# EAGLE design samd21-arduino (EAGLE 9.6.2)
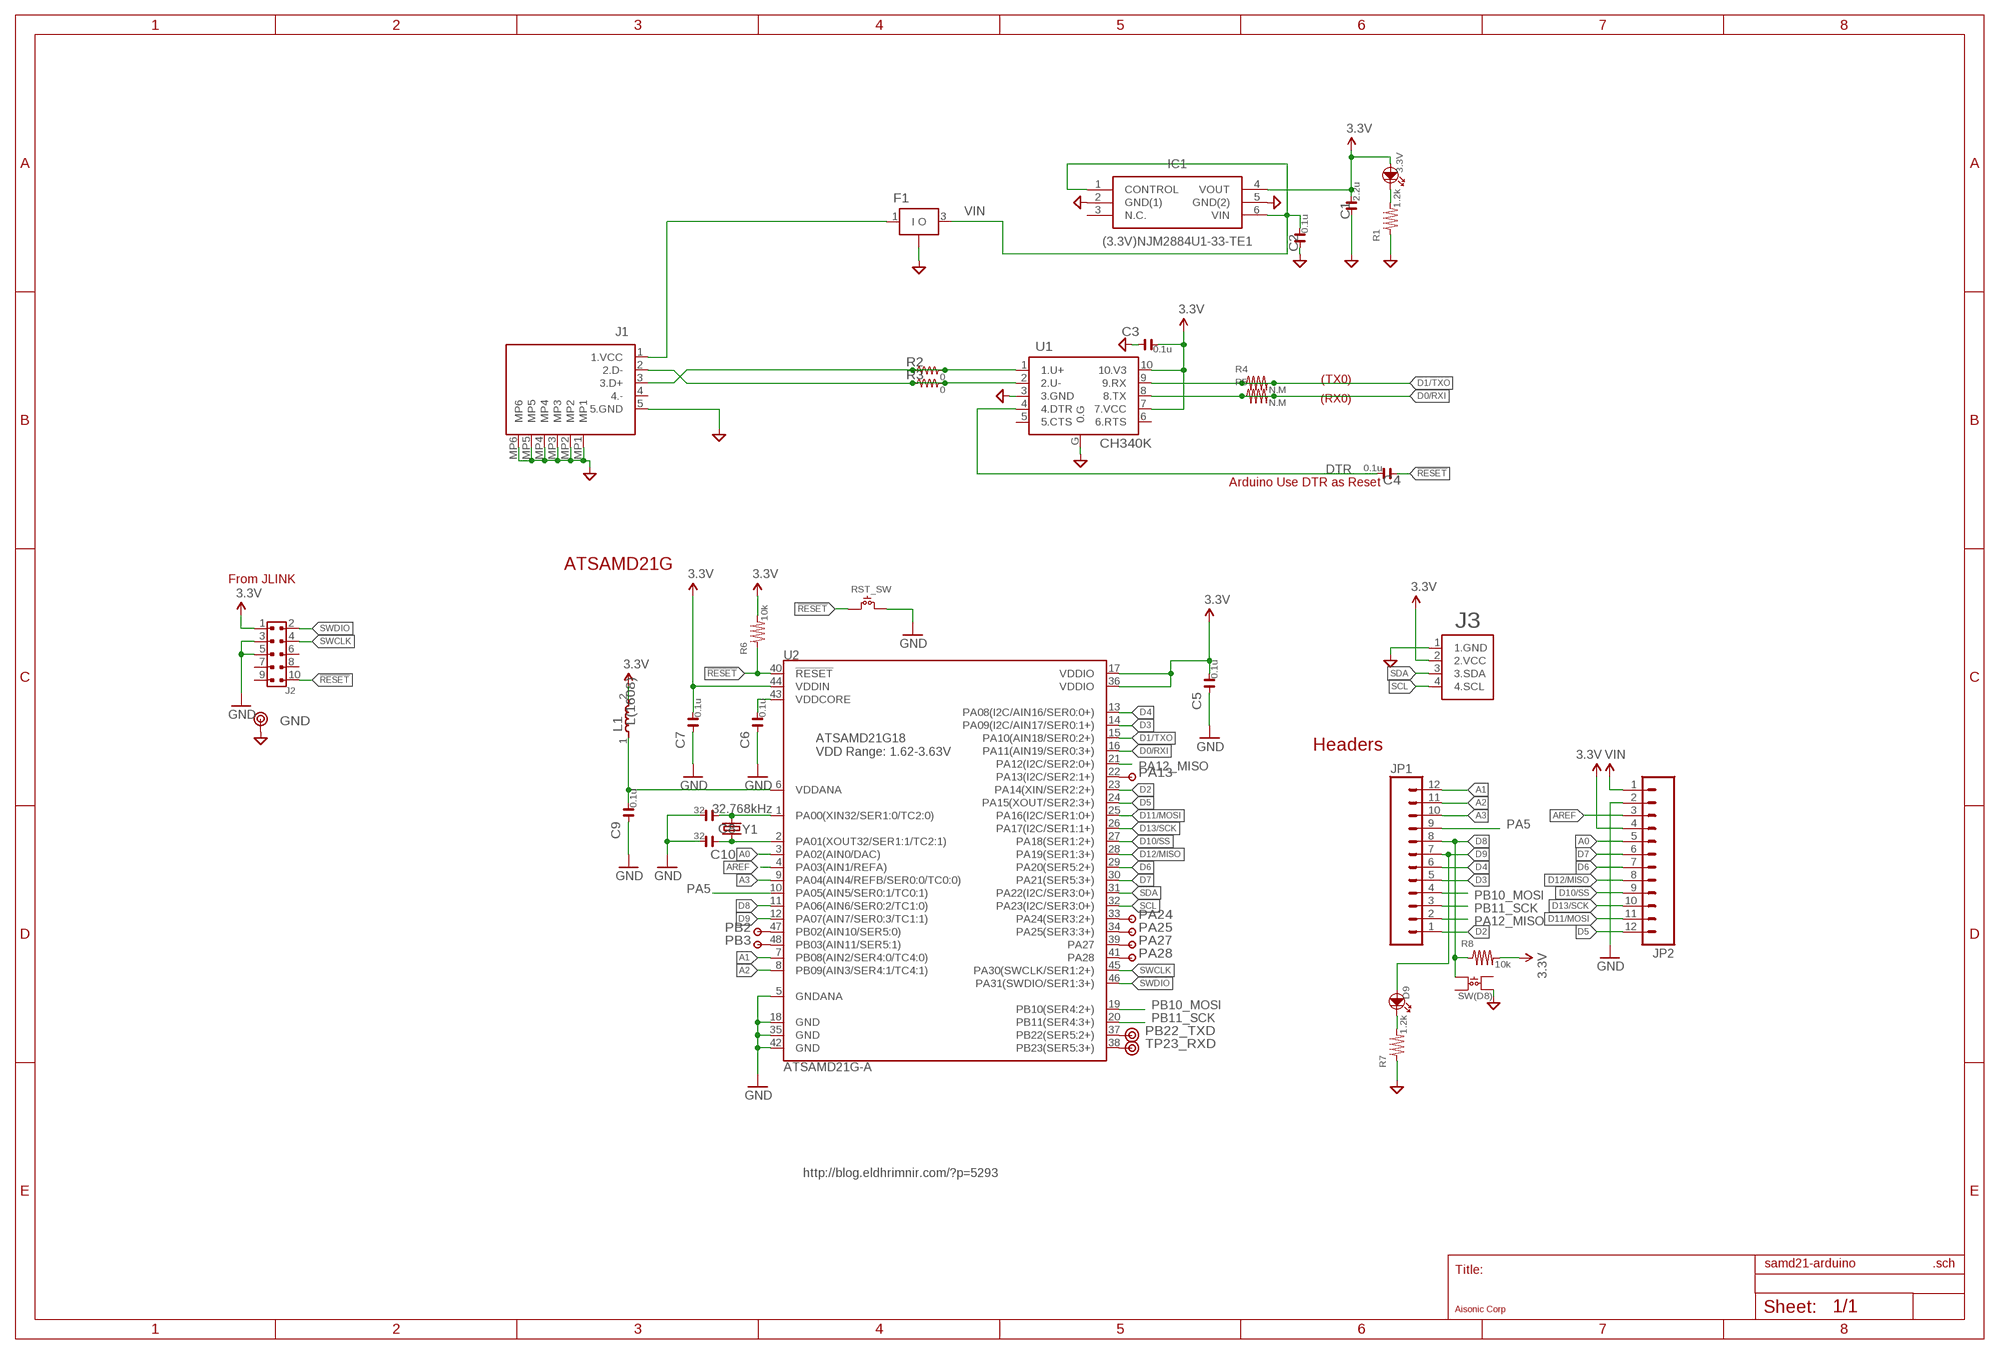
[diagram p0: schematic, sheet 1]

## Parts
3.3V  (PAS)LED[1608]  [1608LED]
C1  2.2u  (PAS)C[1608]  [1608NEW]
C2  0.1u  (PAS)C[1608]  [1608NEW]
C3  0.1u  (PAS)C[1608]  [1608NEW]
C4  0.1u  (PAS)C[1608]  [1608NEW]
C5  0.1u  (PAS)C[1608]  [1608NEW]
C6  0.1u  (PAS)C[1608]  [1608NEW]
C7  0.1u  (PAS)C[1608]  [1608NEW]
C8  32  (PAS)C[1608]  [1608NEW]
C9  0.1u  (PAS)C[1608]  [1608NEW]
C10  32  (PAS)C[1608]  [1608NEW]
D9  (PAS)LED[1608]  [1608LED]
F1  (EMI-FIL)NFM21PC(2012)  [EMIFILL]
FRAME1  (!)A3L-LOC  [D3LOGO-PAC]
GND  TP-HOLE  [TP-HOLE]
IC1  (3.3V)NJM2884U1-33-TE1  [SOT-89-5-1]
J1  (USB)USB-MICRO(ZX62-B-5PA_33)  [ZX62B5PA33]
J2  ARMJTAG10PINSTRAIT  [JTAG_HALFPITCH]
J3  GROVE-I2C  [GROVE-4P]
JP1  M12NO_SILK  [1X12_NO_SILK]
JP2  M12NO_SILK  [1X12_NO_SILK]
L1  L(1608)  [1608NEW]
PA13  TP  [TP-SQUARE]
PA24  TP  [TP-SQUARE]
PA25  TP  [TP-SQUARE]
PA27  TP  [TP-SQUARE]
PA28  TP  [TP-SQUARE]
PB2  TP  [TP-SQUARE]
PB3  TP  [TP-SQUARE]
PB22_TXD  TP-HOLE  [TP-HOLE]
R1  1.2k  (PAS)R[1608]  [1608NEW]
R2  0  R(1005)  [1005]
R3  0  R(1005)  [1005]
R4  N.M  (PAS)R[1608]  [1608NEW]
R5  N.M  (PAS)R[1608]  [1608NEW]
R6  10k  (PAS)R[1608]  [1608NEW]
R7  1.2k  (PAS)R[1608]  [1608NEW]
R8  10k  (PAS)R[1608]  [1608NEW]
RST_SW  (SW)RST_SW(TVAF06)  [TVAF06]
SW(D8)  (SW)USER_SW(AKIDUKI)  [SKRPACE010-PAC]
TP23_RXD  TP-HOLE  [TP-HOLE]
U1  CH340K  (USB)CH340K  [ESSOP10]
U2  ATSAMD21G-A  [TQFP-48]
Y1  32.768kHz  CRYSTAL3.2X1.5MM  [CRYSTAL-SMD-3.2X1.5MM]

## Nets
3.3V: 3.3V.1(+) C1.2 C3.2 C5.2 C7.2 IC1.4(VOUT) J2.1 J3.2(2.VCC) JP2.4 L1.2 R6.2 R8.2 U1.7(7.VCC) U1.10(10.V3) U2.17(VDDIO) U2.36(VDDIO) U2.44(VDDIN)
!RESET: C4.1 J2.10 R6.1 RST_SW.P$1 U2.40(!RESET!)
A0: JP2.5 U2.3(PA02(AIN0/DAC))
A1: JP1.12 U2.7(PB08(AIN2/SER4:0/TC4:0))
A2: JP1.11 U2.8(PB09(AIN3/SER4:1/TC4:1))
A3: JP1.10 U2.9(PA04(AIN4/REFB/SER0:0/TC0:0))
AREF: JP2.3 U2.4(PA03(AIN1/REFA))
D0/RXI: R5.1 R5.2 U1.8(8.TX) U2.16(PA11(AIN19/SER0:3+))
D1/TXO: R4.1 R4.2 U1.9(9.RX) U2.15(PA10(AIN18/SER0:2+))
D2: JP1.1 U2.23(PA14(XIN/SER2:2+))
D3: JP1.5 U2.14(PA09(I2C/AIN17/SER0:1+))
D4: JP1.6 U2.13(PA08(I2C/AIN16/SER0:0+))
D5: JP2.12 U2.24(PA15(XOUT/SER2:3+))
D6: JP2.7 U2.29(PA20(SER5:2+))
D7: JP2.6 U2.30(PA21(SER5:3+))
D8: JP1.8 R8.1 SW(D8).1 U2.11(PA06(AIN6/SER0:2/TC1:0))
D9: D9.1(+) JP1.7 U2.12(PA07(AIN7/SER0:3/TC1:1))
D10/SS: JP2.9 U2.27(PA18(SER1:2+))
D11/MOSI: JP2.11 U2.25(PA16(I2C/SER1:0+))
D12/MISO: JP2.8 U2.28(PA19(SER1:3+))
D13/SCK: JP2.10 U2.26(PA17(I2C/SER1:1+))
DTR: C4.2 U1.4(4.DTR)
GND: C1.1 C2.1 C3.1 C5.1 C6.1 C7.1 C8.2 C9.1 C10.2 F1.2(G) GND.1 IC1.2(GND(1)) IC1.5(GND(2)) J1.5(5.GND) J1.MP1 J1.MP2 J1.MP3 J1.MP4 J1.MP5 J1.MP6 J2.3 J2.5 J3.1(1.GND) JP2.2 R1.1 R7.1 RST_SW.P$2 SW(D8).4 U1.3(3.GND) U1.G(0.G) U2.5(GNDANA) U2.18(GND) U2.35(GND) U2.42(GND)
N$1: PA24.1 U2.33(PA24(SER3:2+))
N$2: C8.1 U2.1(PA00(XIN32/SER1:0/TC2:0)) Y1.P$2
N$3: PA25.1 U2.34(PA25(SER3:3+))
N$4: C10.1 U2.2(PA01(XOUT32/SER1:1/TC2:1)) Y1.P$1
N$5: PA27.1 U2.39(PA27)
N$6: PA28.1 U2.41(PA28)
N$7: D9.2(-) R7.2
N$9: PB22_TXD.1 U2.37(PB22(SER5:2+))
N$10: TP23_RXD.1 U2.38(PB23(SER5:3+))
N$11: PA13.1 U2.22(PA13(I2C/SER2:1+))
N$14: 3.3V.2(-) R1.2
N$15: J1.3(3.D+) R2.1 R2.2 U1.1(1.U+)
N$16: J1.2(2.D-) R3.1 R3.2 U1.2(2.U-)
N$17: PB3.1 U2.48(PB03(AIN11/SER5:1))
N$18: PB2.1 U2.47(PB02(AIN10/SER5:0))
PA5: JP1.9 U2.10(PA05(AIN5/SER0:1/TC0:1))
PA12_MISO: JP1.2 U2.21(PA12(I2C/SER2:0+))
PB10_MOSI: JP1.4 U2.19(PB10(SER4:2+))
PB11_SCK: JP1.3 U2.20(PB11(SER4:3+))
SCL: J3.4(4.SCL) U2.32(PA23(I2C/SER3:0+))
SDA: J3.3(3.SDA) U2.31(PA22(I2C/SER3:0+))
SWCLK: J2.4 U2.45(PA30(SWCLK/SER1:2+))
SWDIO: J2.2 U2.46(PA31(SWDIO/SER1:3+))
VBUS5V1: F1.1(I) J1.1(1.VCC)
VDDANA: C9.2 L1.1 U2.6(VDDANA)
VDDCORE: C6.2 U2.43(VDDCORE)
VIN: C2.2 F1.3(O) IC1.1(CONTROL) IC1.6(VIN) JP2.1
Unconnected: IC1.3(N.C.) J1.4(4.-) J2.6 J2.7 J2.8 J2.9 SW(D8).2 SW(D8).3 U1.5(5.CTS) U1.6(6.RTS)

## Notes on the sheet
- (TX0)
- (RX0)
- Arduino Use DTR as Reset
- ATSAMD21G
- From JLINK
- Headers
- ATSAMD21G18
  VDD Range: 1.62-3.63V
- http://blog.eldhrimnir.com/?p=5293

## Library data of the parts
3.3V D9 = myEagleParts8:(PAS)LED[1608]
C1-C10 = myEagleParts8:(PAS)C[1608]
F1 = myEagleParts8:(EMI-FIL)NFM21PC(2012)
FRAME1 = myEagleParts8:(!)A3L-LOC: FRAME
GND PB22_TXD TP23_RXD = myEagleParts8:TP-HOLE
IC1 = myEagleParts8:(3.3V)NJM2884U1-33-TE1: Low Dropout Voltage Regulator New Japan Radio NJM2884U1-33-TE1, LDO Voltage Regulator, 0.65A, 3.3 V 1%, 5-Pin SOT-89 Source: Datasheet; DESCRIPTION: Low Dropout Voltage Regulator New Japan Radio NJM2884U1-33-TE1, LDO Voltage Regulator, 0.65A, 3.3 V 1%, 5-Pin SOT-89; HEIGHT: mm; MANUFACTURER_NAME: New Japan Radio; MANUFACTURER_PART_NUMBER: NJM2884U1-33-TE1; RS_PART_NUMBER: 7139366P; SUPPLIER_NAME: RS
J1 = myEagleParts8:(USB)USB-MICRO(ZX62-B-5PA_33): USB Connectors MICRO B RECEPT RA SMT BTTM MNT Source: Datasheet; DESCRIPTION: USB Connectors MICRO B RECEPT RA SMT BTTM MNT; HEIGHT: 3mm; MANUFACTURER_NAME: Hirose; MANUFACTURER_PART_NUMBER: ZX62-B-5PA(33); RS_PART_NUMBER: 1362267; RS_PRICE-STOCK: http://uk.rs-online.com/web/p/products/1362267
J2 = myEagleParts8:ARMJTAG10PIN
J3 = myEagleParts8:GROVE-I2C
JP1 JP2 = SparkFun-Connectors:M12: Header 12 Standard 12-pin 0.1" header. Use with straight break away headers (SKU : PRT-00116), right angle break away headers (PRT-00553), swiss pins (PRT-00743), machine pins (PRT-00117), and female headers (PRT-00115).
L1 = myEagleParts8:L(1608)
PA13 PA24 PA25 PA27 PA28 PB2 PB3 = myEagleParts8:TP
R1 R4-R8 = myEagleParts8:(PAS)R[1608]
R2 R3 = myEagleParts8:R(1005)
RST_SW = myEagleParts8:(SW)RST_SW(TVAF06)
SW(D8) = myEagleParts8:(SW)USER_SW(AKIDUKI): http://akizukidenshi.com/catalog/g/gP-06185/
U1 = myEagleParts8:(USB)CH340K
U2 = samd21-temp:ATSAMD21G: Atmel SAMD21G SMART ARM-Based Microcontroller The Atmel ® | SMART ™ SAM D21 is a series of low-power microcontrollers using the 32-bit ARM ® Cortex ® -M0+ processor, and ranging from 32- to 64-pins with up to 256KB Flash and 32KB of SRAM. The SAM D21 devices operate at a maximum frequency of 48MHz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; PROD_ID: IC-13064
Y1 = samd21-temp:CRYSTAL: Various standard crystals. Proven footprints.; PROD_ID: XTAL-13062

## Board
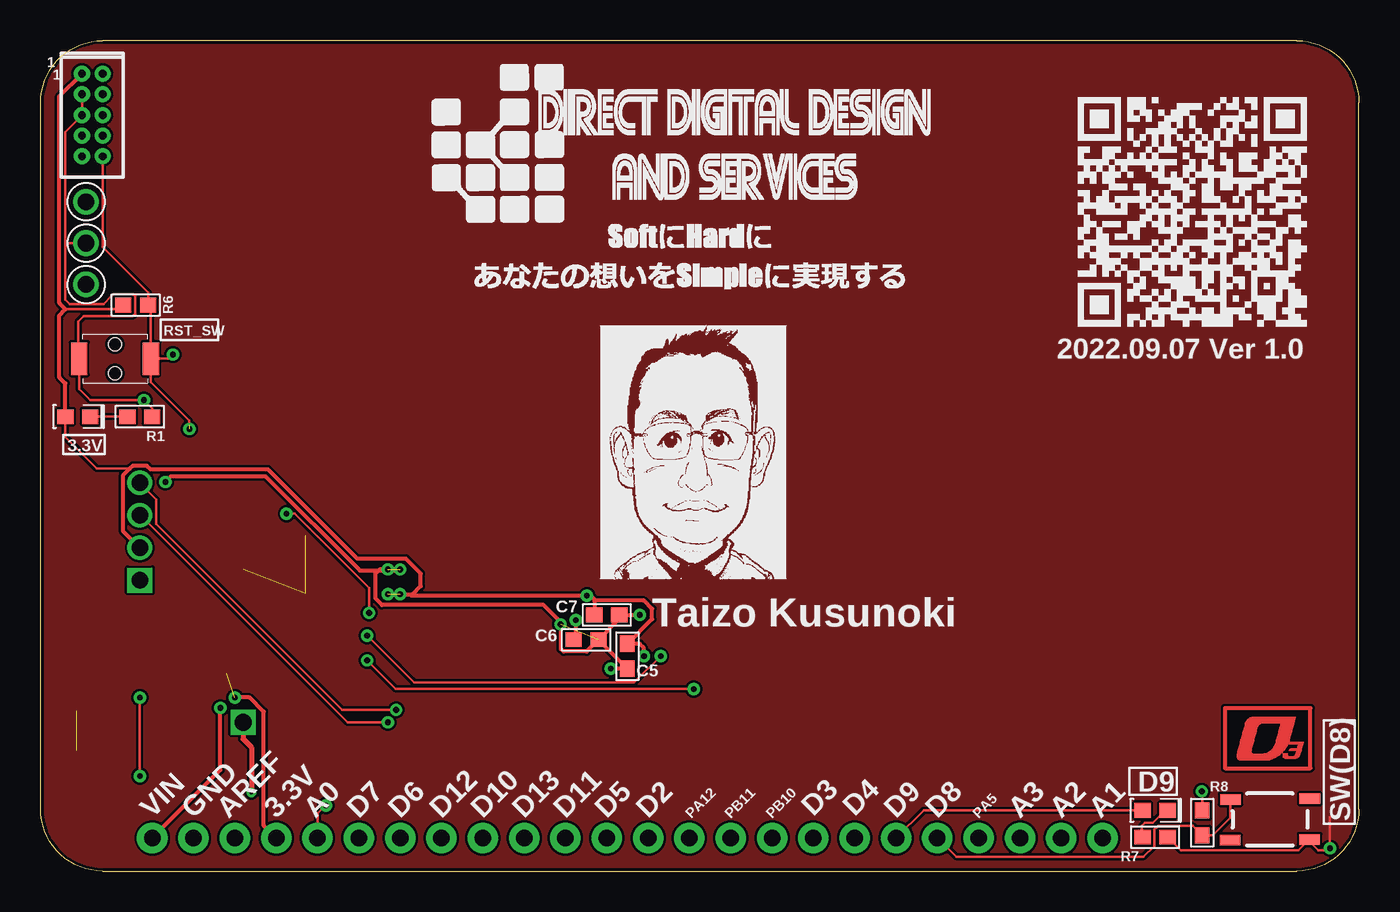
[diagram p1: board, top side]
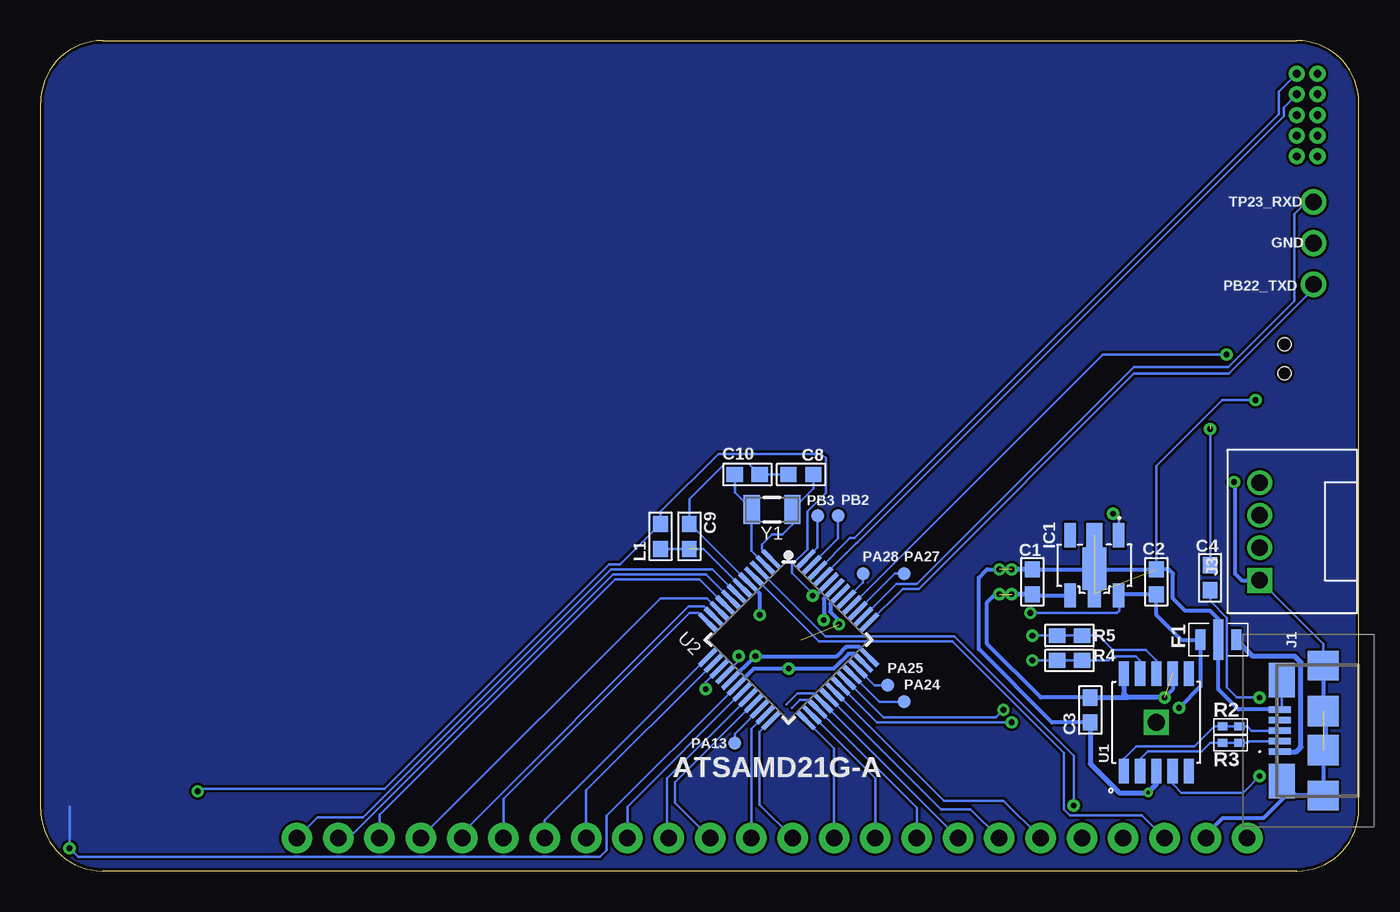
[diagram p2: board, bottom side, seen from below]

Size 81.03 x 51.05 mm. Coordinates in mm from the lower left corner, seen from the top.
Outline: 0,3.56 0,47.24 arc-90 3.81,51.05 77.22,51.05 arc-90 81.03,47.24 81.03,3.81 arc-90 77.22,0 3.81,0 arc-90 0,3.81
Copper layers (1*16): Top 0.035mm / dielectric 1.5mm / Bottom 0.035mm
Design rules "PCBGoGo": minimum track width 6mil, minimum drill 0.2mm, track to track 6mil, track to pad 6mil, pad to pad 6mil, via to via 6mil, smd to smd 6mil, copper to edge 0.2mm, drill to drill 6mil, minimum pad ring 10mil, minimum via ring 8mil, stop-mask expansion 4mil, vias tented up to drill 0mil, thermal gap 10mil

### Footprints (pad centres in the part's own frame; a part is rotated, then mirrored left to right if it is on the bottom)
1608LED = smd 1 x 0.9: 1 -0.766,0; 2 0.766,0
1608NEW = smd 1 x 0.9: 1 -0.766,0; 2 0.766,0
EMIFILL = smd 0.6 x 1.25: 1 -1.1,0; 3 1.1,0 | smd 0.6 x 2.5: 2 0,0
TP-HOLE = drill 1.016 pad 1.575: 1 0,0
SOT-89-5-1 = smd 0.7 x 1.5: 1 -1.5,-1.85; 3 1.5,-1.85; 4 1.5,1.85; 6 -1.5,1.85 | smd 1 x 1.5: 2 0,-1.85 | smd 0.8 x 1.5: 5 0,1.85 | smd 1.5 x 2.6: 7 0,0.2
ZX62B5PA33 = smd 0.4 x 1.35: 1 -1.3,2.325; 2 -0.65,2.325; 3 0,2.325; 4 0.65,2.325; 5 1.3,2.325 | smd 1.8 x 1.9: MP1 -4,-0.35; MP2 4,-0.35 | smd 2.1 x 1.6: MP3 -3.1,2.2; MP4 3.1,2.2 | smd 1.9 x 1.9: MP5 -1.2,-0.35; MP6 1.2,-0.35
JTAG_HALFPITCH = drill 0.483 pad 0.61: 1 0,0; 2 1.27,0; 3 0,-1.27; 4 1.27,-1.27; 5 0,-2.54; 6 1.27,-2.54; 7 0,-3.81; 8 1.27,-3.81; 9 0,-5.08; 10 1.27,-5.08
GROVE-4P = drill 1.016 square: 1 6,0 | drill 1.016: 2 4,0; 3 2,0; 4 0,0
1X12_NO_SILK = drill 1.016 pad 1.88: 1 0,0; 2 2.54,0; 3 5.08,0; 4 7.62,0; 5 10.16,0; 6 12.7,0; 7 15.24,0; 8 17.78,0; 9 20.32,0; 10 22.86,0; 11 25.4,0; 12 27.94,0
TP-SQUARE = smd 0.8 x 0.8: 1 0,0
1005 = smd 0.6 x 0.5: 1 -0.508,0; 2 0.519,0
TVAF06 = smd 2 x 1: P$1 0,2.2; P$2 0,-2.2 | hole 0.8: -0.9,0; 0.9,0
SKRPACE010-PAC = smd 1.27 x 0.635: 1 -2.427,1.227; 2 -2.45,-1.277; 3 2.45,1.277; 4 2.427,-1.227
ESSOP10 = smd 1.5 x 0.635: 1 -3,2; 2 -3,1; 3 -3,0; 4 -3,-1; 5 -3,-2; 6 3,-2; 7 3,-1; 8 3,0; 9 3,1; 10 3,2 | drill 1.016 square: G 0,0
TQFP-48 = smd 1.5 x 0.28: 1 -4.25,2.75; 2 -4.25,2.25; 3 -4.25,1.75; 4 -4.25,1.25; 5 -4.25,0.75; 6 -4.25,0.25; 7 -4.25,-0.25; 8 -4.25,-0.75; 9 -4.25,-1.25; 10 -4.25,-1.75; 11 -4.25,-2.25; 12 -4.25,-2.75; 25 4.25,-2.75; 26 4.25,-2.25; 27 4.25,-1.75; 28 4.25,-1.25; 29 4.25,-0.75; 30 4.25,-0.25; 31 4.25,0.25; 32 4.25,0.75; 33 4.25,1.25; 34 4.25,1.75; 35 4.25,2.25; 36 4.25,2.75 | smd 0.28 x 1.5: 13 -2.75,-4.25; 14 -2.25,-4.25; 15 -1.75,-4.25; 16 -1.25,-4.25; 17 -0.75,-4.25; 18 -0.25,-4.25; 19 0.25,-4.25; 20 0.75,-4.25; 21 1.25,-4.25; 22 1.75,-4.25; 23 2.25,-4.25; 24 2.75,-4.25; 37 2.75,4.25; 38 2.25,4.25; 39 1.75,4.25; 40 1.25,4.25; 41 0.75,4.25; 42 0.25,4.25; 43 -0.25,4.25; 44 -0.75,4.25; 45 -1.25,4.25; 46 -1.75,4.25; 47 -2.25,4.25; 48 -2.75,4.25
CRYSTAL-SMD-3.2X1.5MM = smd 1 x 1.8: P$1 -1.25,0; P$2 1.25,0

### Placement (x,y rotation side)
3.3V  2.29,27.94 0 top
C1  20.07,17.78 270 bottom
C2  12.45,17.78 270 bottom
C3  16.51,9.91 90 bottom
C4  9.14,18.03 270 bottom
C5  36.07,13.21 90 top
C6  33.53,14.22 180 top
C7  34.8,15.75 180 top
C8  34.29,24.38 180 bottom
C9  41.15,20.57 270 bottom
C10  37.59,24.38 0 bottom
D9  68.5,3.73 0 top
F1  8.64,14.22 180 bottom
FRAME1  72.8,6.38 0 top
GND  2.79,38.61 0 top
IC1  16.26,18.8 180 bottom
J1  2.54,8.64 90 bottom
J2  2.54,49.02 0 top
J3  6.1,23.88 270 bottom
JP1  37.34,2.03 0 top
JP2  6.86,2.03 0 top
L1  42.93,20.57 90 bottom
PA13  38.35,7.87 0 bottom
PA24  27.94,10.41 0 bottom
PA25  28.96,11.43 0 bottom
PA27  27.94,18.29 0 bottom
PA28  30.48,18.29 0 bottom
PB2  32,21.84 0 bottom
PB3  33.27,21.84 0 bottom
PB22_TXD  2.79,36.07 0 top
R1  6.1,27.94 180 top
R2  7.87,8.89 0 bottom
R3  7.87,7.87 0 bottom
R4  17.78,12.95 180 bottom
R5  17.78,14.48 180 bottom
R6  5.84,34.8 180 top
R7  68.5,2.08 180 top
R8  71.4,2.97 90 top
RST_SW  4.57,31.5 270 top
SW(D8)  75.56,3.17 0 top
TP23_RXD  2.79,41.15 0 top
U1  12.45,9.14 90 bottom
U2  35.05,14.22 315 bottom
Y1  36.07,22.23 0 bottom

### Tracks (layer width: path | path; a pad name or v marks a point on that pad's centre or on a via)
3.3V  (via drill 0.35 pad 0.3)  (2 unrouted)
  Top 0.152: R6.2 4.82,34.54 1.52,34.54 | 3.3V.1 1.52,26.67 3.46,24.74 5.49,24.74 | v71.37,4.9 71.4,4.88 R8.2
  Top 0.254: 34.03,16.64 34.03,16.7 33.73,17 33.66,17 v33.58,16.93 33.49,16.93 33.48,16.94 22.78,16.94 22.86,17.02 | 34.03,16.64 C7.2 | v37.08,13.21 37.08,13.72 36.83,13.97 C5.2 37.59,15.5 37.59,16.13 37.08,16.64 34.03,16.64 | J2.1 1.14,47.62 1.14,34.92 1.52,34.54 1.14,34.16 1.14,30.35 1.52,29.98 3.3V.1 | JP2.4 13.72,2.79 13.72,9.79 12.84,10.67 v11.94,10.67 | v21.34,17.02 22.86,17.02 | 22.86,17.02 23.37,17.53 23.37,18.29 22.46,19.2 19.48,19.2 13.98,24.69 6.75,24.69 6.53,24.92 5.67,24.92 5.49,24.74 5.05,24.31 5.05,20.92 J3.2
  Bottom 0.152: 33.58,17.07 v33.58,16.93 | 33.58,17.07 34.85,18.34 34.85,18.84 33.9,19.78 33.9,22.1 32.77,23.24 32.77,25.4 33.02,25.65 39.37,25.65 42.93,22.1 L1.2 45.42,18.85 46.1,18.85 59.89,5.05 71.22,5.05 v71.37,4.9 | 33.58,17.07 33.53,17.02
  Bottom 0.254: U2.44 33.32,17.02 33.53,17.02 | U2.17 37.13,13.21 v37.08,13.21 32.09,13.21 31.52,13.77 30.71,13.77 U2.36 | C1.2 20,16.95 IC1.4 | C3.2 19.56,10.67 22.86,13.97 22.86,16.51 22.36,17.01 v22.09,17.01 | U1.7 11.45,11.16 v11.93,10.67
  Bottom 0.305: C3.2 14.22,10.67 | v11.93,10.67 14.22,10.67 | U1.10 14.45,10.89 14.22,10.67 | C1.2 v22.09,17.01 v22.1,17.02
!RESET  (via drill 0.35 pad 0.3)  (1 unrouted)
  Top 0.152: v8.13,31.75 7.87,31.5 RST_SW.P$1 | RST_SW.P$1 6.77,34.38 6.6,34.54 R6.1 | R6.1 | J2.10 3.81,38.35 6.6,35.56 R6.1 | RST_SW.P$1 6.77,30.06 9.14,27.69 v9.14,27.18
  Bottom 0.152: U2.40 15.75,31.75 v8.13,31.75 | 9.14,27.43 C4.1
A0  (via drill 0.35 pad 0.3)
  Top 0.152: JP2.5 17.02,3.56 17.5,4.04 v17.53,4.04
  Bottom 0.152: U2.3 32.78,14.43 24.87,14.43 17.53,7.08 v17.53,4.04
A1
  Bottom 0.152: U2.7 39.72,18.54 45.97,18.54 61.21,3.3 64.01,3.3 JP1.12
A2
  Bottom 0.152: U2.8 40.13,18.24 45.85,18.24 62.05,2.03 JP1.11
A3
  Bottom 0.152: U2.9 40.53,17.93 45.72,17.93 60.2,3.46 JP1.10
AREF
  Bottom 0.152: U2.4 33.18,14.12 25,14.12 18.13,7.26 18.13,3.78 17.78,3.43 13.34,3.43 JP2.3
BETA_L1
  Top 0.152: 79.25,1.27 79.25,3.3
  pour Top: -2.54,53.34 83.82,53.34 83.82,-2.54 -2.54,-2.54
BETA_L2
  Bottom 0.152: 79.25,1.27 79.25,3.94
  pour Bottom: -5.08,55.88 86.36,55.88 86.36,-5.08 -5.08,-5.08
D0/RXI  (via drill 0.35 pad 0.3)
  Top 0.152: v20.07,14.48 22.96,11.59 36.49,11.59 38.11,13.21 v38.11,13.22
  Bottom 0.152: U1.8 12.45,12.95 13.08,13.59 15.11,13.59 16,14.48 R5.1 R5.2 v20.07,14.48 | v38.11,13.22 38.1,13.21 38.1,12.94 U2.16
D1/TXO  (via drill 0.35 pad 0.3)
  Top 0.152: v40.15,11.19 21.83,11.19 v20.07,12.95
  Bottom 0.152: U1.9 13.45,12.94 13.72,13.21 15.11,13.21 15.37,12.95 R4.1 R4.2 v20.07,12.95 | U2.15 40.15,11.6 v40.15,11.19
D2
  Bottom 0.152: U2.23 37.34,8.76 JP1.1
D3
  Bottom 0.152: JP1.5 47.5,4.96 U2.14
D4
  Bottom 0.152: JP1.6 50.04,3.13 U2.13
D5
  Bottom 0.152: U2.24 36.83,8.56 36.83,4.06 JP2.12
D6
  Bottom 0.152: U2.29 25.7,3.81 23.88,3.81 JP2.7
D7
  Bottom 0.152: U2.30 25.5,4.32 21.84,4.32 JP2.6
D8
  Top 0.152: SW(D8).1 73.14,3.29 72.06,2.21 R8.1 70.81,2.79 68.7,2.79 68.47,2.56 68.47,1.54 67.79,0.86 56.29,0.86 JP1.8
  Bottom 0.152: U2.11 40.27,16.26 41.2,16.26 55.12,2.34 JP1.8
D9
  Top 0.152: JP1.7 54.28,3.73 D9.1
  Bottom 0.152: U2.12 40.59,15.88 41.15,15.88 52.58,4.45 JP1.7
D10/SS
  Bottom 0.152: 34.85,10.03 34.34,10.54 33.84,10.54 U2.27 27.18,3.88 JP2.9
D11/MOSI
  Bottom 0.152: JP2.11 32.26,7.54 U2.25
D12/MISO
  Bottom 0.152: 35.18,10.26 34.52,10.92 33.52,10.92 U2.28 24.64,2.04 JP2.8
D13/SCK
  Bottom 0.152: U2.26 29.72,5.71 JP2.10
DTR  (via drill 0.35 pad 0.3)
  Top 0.152: v6.1,5.84 v6.1,10.67
  Bottom 0.152: U1.4 11.45,5.35 10.92,4.83 7.11,4.83 v6.1,5.84 | 8.89,17.27 C4.2 9.14,16.61 8.11,15.57 8.11,11.28 7.49,10.67 v6.1,10.67
GND  (via drill 0.2 pad 0.3, 0.35 pad 0.3)  (5 unrouted)
  Top 0.152: J2.3 J2.5 1.5,45.44 1.5,38.35 | v6.35,28.96 3.05,28.96 2.37,29.63 RST_SW.P$2 2.32,31.55 2.32,33.78 2.66,34.12 5.67,34.12 5.8,34.25 5.8,35.34 5.67,35.48 4.48,35.48 4.35,35.34 3.86,34.85 1.78,34.85 1.5,35.13 1.5,38.35 | v6.35,28.96 6.86,28.44 R1.1 | GND.1 1.75,38.61 1.5,38.35 | v6.35,28.96 | v79.25,1.4 79.12,1.27 78.54,1.27 77.99,1.82 SW(D8).4 77.31,1.27 70.08,1.27 R7.1
  Top 0.254: C6.1 35.56,15.49 C7.1 v36.83,15.75 | C6.1 C5.1 v35.06,12.44 v35.05,12.45 | v7.67,23.92 8.03,24.29 13.81,24.29 19.62,18.48 22.04,18.48 v22.1,18.54 20.83,18.54 20.57,18.29 20.57,16.76 20.98,16.36 30.92,16.36 31.98,15.3 31.98,13.66 32.15,13.49 33.56,13.49 C6.1
  Top 0.305: U1.G 12.45,8.13 12.95,7.62 v12.95,4.83
  Bottom 0.152: C8.2 C10.2 37.51,25.06 38.95,25.06 41.15,22.87 C9.1 41.11,21.34 U2.5 | J1.MP4 4.74,10.06 J1.5 | C2.1 12.45,24.89 8.38,28.96 v6.35,28.96 | 2.19,12.45 2.19,13.97 J3.1 | IC1.5 16.26,17.07 | U2.18 46.23,3.4 46.23,1.27 46.63,0.86 55.6,0.86 55.63,0.89 57.15,0.89 57.17,0.86 78.72,0.86 v79.25,1.4
  Bottom 0.254: J1.5 7.4,9.94 8.64,11.18 F1.2 8.64,15.49 9.14,16 10.67,16 11.43,16.76 11.43,18.29 11.69,18.55 C2.1 C1.1 | U2.35 31.01,13.37 31.36,13.37 32.27,12.45 v35.05,12.45 37.18,12.45 U2.18 | U2.42 32.49,16.44 32.49,15.94 31.95,15.41 v31.95,15.16 | J1.MP2 2.19,12.45 2.19,9.43 2.03,9.27 2.03,7.59 J1.MP5 2.19,4.7 | 2.19,4.7 J1.MP1 4.48,4.64 5.86,3.25 8.38,3.25 9.4,2.23 JP2.2 | J1.MP3 3.9,4.7 2.19,4.7 | C3.1 18.86,9.14 23.37,13.65 23.37,18.03 22.86,18.55 21.84,18.55 | U2.5 36.83,17.06 v36.83,15.75 | v7.67,23.92 7.62,23.88 7.62,18.29 7.21,17.88 J3.1
  Bottom 0.305: C3.1 16.51,6.6 14.73,4.83 v12.95,4.83 12.45,5.33 U1.3 | C1.1 21.84,18.55 v22.09,18.55 v22.1,18.54
  other vias: 21.34,18.54
N$1
  Bottom 0.152: U2.33 29.47,10.41 PA24.1
N$2
  Bottom 0.152: U2.1 36.7,19.76 36.7,20.07 36.07,20.7 35.43,20.7 34.82,21.32 Y1.P$2 33.52,23.52 C8.1
N$3
  Bottom 0.152: U2.34 29.78,11.43 PA25.1
N$4
  Bottom 0.152: U2.2 37.32,19.67 Y1.P$1 38.36,23.27 C10.1
N$5
  Bottom 0.152: U2.39 28.51,18.29 PA27.1
N$6
  Bottom 0.152: U2.41 30.48,17.73 PA28.1
N$7
  Top 0.152: 69.27,3.62 D9.2 69.12,3.73 68.36,2.97 67.87,2.97 67.69,2.79 67.69,2.13 R7.2
N$9
  Bottom 0.152: U2.37 28.03,17.36 27.05,17.36 13.82,30.58 8.01,30.58 2.79,35.8 PB22_TXD.1
N$10
  Bottom 0.152: U2.38 28.43,17.66 27.17,17.66 13.84,30.99 8.03,30.99 3.96,35.05 3.96,40.4 3.21,41.15 TP23_RXD.1
N$11
  Bottom 0.152: U2.22 38.35,8.45 PA13.1
N$14
  Top 0.152: R1.2 3.3V.2
N$15
  Bottom 0.152: J1.3 6.6,8.64 6.86,8.89 R2.2 R2.1 8.89,8.89 10.11,7.67 13.66,7.67 14.45,6.89 U1.1
N$16
  Bottom 0.152: J1.2 6.75,7.99 6.86,7.87 R3.2 R3.1 9.14,7.87 9.65,7.37 12.95,7.37 13.45,6.87 U1.2
N$17
  Bottom 0.152: U2.48 33.27,19.89 PB3.1
N$18
  Bottom 0.152: U2.47 32,20.45 PB2.1
PA5
  Bottom 0.152: U2.10 40.07,16.76 42.93,16.76 JP1.9
PA12_MISO
  Bottom 0.152: U2.21 42.04,5.47 42.04,4.2 JP1.2
PB10_MOSI
  Bottom 0.152: JP1.4 44.96,3.96 U2.19
PB11_SCK
  Bottom 0.152: U2.20 42.53,5.69 42.53,2.14 JP1.3
SCL  (via drill 0.35 pad 0.3)
  Top 0.152: v21.84,9.91 18.54,9.91 7.11,21.34 7.11,22.86 J3.4
  Bottom 0.152: U2.32 29.22,9.45 22.3,9.45 v21.84,9.91
SDA  (via drill 0.35 pad 0.3)
  Top 0.152: v21.34,9.14 18.87,9.14 6.14,21.88 J3.3
  Bottom 0.152: v21.34,9.14 29.62,9.14 U2.31
SWCLK
  Bottom 0.152: U2.45 31.5,19.55 31.5,19.56 30.88,20.17 30.86,20.17 4.62,46.42 4.62,46.95 J2.4
SWDIO
  Bottom 0.152: U2.46 31.28,20.48 30.99,20.48 4.92,46.55 4.92,47.91 J2.2
VBUS5V1
  Bottom 0.305: J1.1 3.84,7.34 3.56,7.62 3.56,12.83 3.93,13.21 6.52,13.21 F1.1
VDDANA  (1 unrouted)
  Bottom 0.152: U2.6 40.29,19.81 40.64,19.81 | C9.2 L1.1
VDDCORE  (via drill 0.35 pad 0.3)
  Top 0.152: 32.89,14.36 C6.2
  Top 0.254: v32.89,15.42 32.89,14.36
  Bottom 0.254: U2.43 32.89,16.74 v32.89,15.42
VIN  (via drill 0.35 pad 0.3)
  Top 0.152: v15.11,21.97 15.63,21.97 20.19,17.4 v20.19,15.88
  Top 0.254: JP2.1 11.05,6.22 v11.05,10.03
  Bottom 0.152: IC1.1 14.76,21.61 v15.11,21.97 | 14.73,17.01 14.73,16 14.86,15.88 v20.19,15.88
  Bottom 0.254: 14.69,17.01 14.73,17.01 | 14.69,17.01 C2.2 12.45,15.75 10.92,14.22 F1.3 9.74,11.35 v11.05,10.03 | 14.69,17.01 IC1.6

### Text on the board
tPlace: 1 | 2022.09.07 Ver 1.0 | Taizo Kusunoki | VIN | GND | AREF | 3.3V | A0 | D7 | D6 | D12 | D10 | D13 | D11 | D5 | D2 | PA12 | PB11 | PB10 | D3 | D4 | D9 | D8 | PA5 | A3 | A2 | A1
bPlace: ATSAMD21G-A

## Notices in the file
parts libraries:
SparkFun-Connectors: Licensing: Creative Commons ShareAlike 4.0 International - https://creativecommons.org/licenses/by-sa/4.0
